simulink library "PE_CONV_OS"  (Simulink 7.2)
settings: Solver=ode45  SolverMode=SingleTasking  StartTime=0.0  StopTime=10.0  RelTol=1e-3
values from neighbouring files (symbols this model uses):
  C = 10e-3*1    (= 0.01)    [INIT_B6_2L_3Ph_IGBT_OS.m]    (also in INIT_B6_3L_3Ph_IGBT_OS.m; INIT_MMC_100L.m = 0.005; INIT_MMC_200L.m = 0.005; INIT_MMC_20L.m)
  FS = 900    [INIT_B6_2L_3Ph_IGBT_OS.m]    (also in INIT_B6_3L_3Ph_IGBT_OS.m; INIT_PWM_2L.m = 1000; INIT_PWM_3L.m = 1000; INIT_PWM_Con.m = 1000)
  LN = 2e-3    (= 0.002)    [INIT_PWM_2L.m]    (also in INIT_PWM_3L.m; INIT_PWM_Con.m; INIT_MMC_100L.m = 0.025; INIT_MMC_200L.m = 0.025)
  LS = 1e-3    (= 0.001)    [INIT_B6_2L_3Ph_IGBT_OS.m]    (also in INIT_B6_3L_3Ph_IGBT_OS.m; INIT_MMC_100L.m = 0.025; INIT_MMC_200L.m = 0.025; INIT_MMC_20L.m = 0.0025)
  LT = LN    (= 0.025)    [INIT_MMC_100L.m]    (also in INIT_MMC_200L.m; INIT_MMC_20L.m = 0.002; INIT_MMC_400L.m)
  Nc = 100    [INIT_MMC_100L.m]    (also in INIT_MMC_200L.m = 200; INIT_MMC_20L.m = 20; INIT_MMC_400L.m = 400)
  NT = sqrt(3)*340/400    [INIT_MMC_100L.m]    (also in INIT_MMC_200L.m; INIT_MMC_20L.m = sqrt(3); INIT_MMC_400L.m)
  Rg = 1e-3    (= 0.001)    [INIT_MMC_100L.m]    (also in INIT_MMC_200L.m; INIT_MMC_20L.m; INIT_MMC_400L.m)
  RN = 0.1    [INIT_PWM_2L.m]    (also in INIT_PWM_3L.m; INIT_PWM_Con.m; INIT_MMC_100L.m; INIT_MMC_200L.m)
  RT = RN    (= 0.1)    [INIT_MMC_100L.m]    (also in INIT_MMC_200L.m; INIT_MMC_20L.m; INIT_MMC_400L.m)
  UC0 = 600    [INIT_B6_2L_3Ph_IGBT_OS.m]    (also in INIT_B6_3L_3Ph_IGBT_OS.m = 500; INIT_MMC_100L.m = 6800; INIT_MMC_200L.m = 3400; INIT_MMC_20L.m = 5000)
undefined symbols (not defined in the file or in its folder): A, DT, FT, L, O1, O2, PHT, T, Td
libraries: simulink_extras x2
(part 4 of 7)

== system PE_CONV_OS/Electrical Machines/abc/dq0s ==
  a : Inport  OutDataType=sfix(16)  OutScaling=2^0
  b : Inport  Port=2  OutDataType=sfix(16)  OutScaling=2^0
  c : Inport  Port=3  OutDataType=sfix(16)  OutScaling=2^0
  Demux : Demux  Outputs=3
  K : Gain  Gain="2/3*[1   -.5   -.5;  0   sqrt(3)/2   -sqrt(3)/2;  .5    .5    .5]"  Multiplication=Matrix(K*u)  ParameterDataType=sfix(16)  ParameterScaling=2^0  OutDataType=sfix(16)  OutScaling=2^0
  Mux : Mux  Inputs=3
  d : Outport
  q : Outport  Port=2
  0 : Outport  Port=3
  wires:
  c/1 -> Mux/3
  b/1 -> Mux/2
  K/1 -> Demux/1
  Mux/1 -> K/1
  a/1 -> Mux/1
  Demux/1 -> d/1
  Demux/2 -> q/1
  Demux/3 -> 0/1

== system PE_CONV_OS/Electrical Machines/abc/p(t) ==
  Uabc : Inport
  Iabc : Inport  Port=2
  Fcn : Fcn  Expr=u(1)*u(4) + u(2)*u(5) + u(3)*u(6)
  Mux : Mux  Inputs=2
  Pt : Outport
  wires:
  Uabc/1 -> Mux/1
  Iabc/1 -> Mux/2
  Mux/1 -> Fcn/1
  Fcn/1 -> Pt/1

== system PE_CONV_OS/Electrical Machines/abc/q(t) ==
  Uabc : Inport
  Iabc : Inport  Port=2
  Fcn : Fcn  Expr="(  (u(2) - u(3))* u(4) + (u(3) - u(1))* u(5) + (u(1) - u(2))* u(6)  )/ sqrt(3)"
  Mux : Mux  Inputs=2
  qt : Outport
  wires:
  Uabc/1 -> Mux/1
  Iabc/1 -> Mux/2
  Mux/1 -> Fcn/1
  Fcn/1 -> qt/1

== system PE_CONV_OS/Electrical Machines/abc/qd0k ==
  a : Inport  OutDataType=sfix(16)  OutScaling=2^0
  b : Inport  Port=2  OutDataType=sfix(16)  OutScaling=2^0
  c : Inport  Port=3  OutDataType=sfix(16)  OutScaling=2^0
  th : Inport  Port=4  OutDataType=sfix(16)  OutScaling=2^0
  Demux : Demux  Outputs=3
  Fcn : Fcn  Expr=u(1)*cos(u(3)) - u(2)*sin(u(3))
  Fcn1 : Fcn  Expr=u(1)*sin(u(3)) + u(2)*cos(u(3))
  K : Gain  Gain="2/3*[1   -.5   -.5;  0   -sqrt(3)/2   sqrt(3)/2;  .5    .5    .5]"  Multiplication=Matrix(K*u)  ParameterDataType=sfix(16)  ParameterScaling=2^0  OutDataType=sfix(16)  OutScaling=2^0
  Mux : Mux  Inputs=3
  Mux1 : Mux  Inputs=3
  qk : Outport
  dk : Outport  Port=2
  0k : Outport  Port=3
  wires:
  Demux/2 -> Mux1/2
  Demux/1 -> Mux1/1
  Demux/3 -> 0k/1
  th/1 -> Mux1/3
  Fcn1/1 -> dk/1
  Fcn/1 -> qk/1
  Mux1/1 -> Fcn/1, Fcn1/1
  a/1 -> Mux/1
  Mux/1 -> K/1
  K/1 -> Demux/1
  b/1 -> Mux/2
  c/1 -> Mux/3

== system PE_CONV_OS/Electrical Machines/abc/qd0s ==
  a : Inport  OutDataType=sfix(16)  OutScaling=2^0
  b : Inport  Port=2  OutDataType=sfix(16)  OutScaling=2^0
  c : Inport  Port=3  OutDataType=sfix(16)  OutScaling=2^0
  Demux : Demux  Outputs=3
  K : Gain  Gain="2/3*[1   -.5   -.5;  0   -sqrt(3)/2   sqrt(3)/2;  .5    .5    .5]"  Multiplication=Matrix(K*u)  ParameterDataType=sfix(16)  ParameterScaling=2^0  OutDataType=sfix(16)  OutScaling=2^0
  Mux : Mux  Inputs=3
  q : Outport
  d : Outport  Port=2
  0 : Outport  Port=3
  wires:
  Demux/3 -> 0/1
  Demux/2 -> d/1
  Demux/1 -> q/1
  a/1 -> Mux/1
  Mux/1 -> K/1
  K/1 -> Demux/1
  b/1 -> Mux/2
  c/1 -> Mux/3

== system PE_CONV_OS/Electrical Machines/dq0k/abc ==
  dk : Inport  OutDataType=sfix(16)  OutScaling=2^0
  qk : Inport  Port=2  OutDataType=sfix(16)  OutScaling=2^0
  0k : Inport  Port=3  OutDataType=sfix(16)  OutScaling=2^0
  th : Inport  Port=4  OutDataType=sfix(16)  OutScaling=2^0
  Demux : Demux  Outputs=3
  Fcn : Fcn  Expr=u(1)*cos(u(3)) - u(2)*sin(u(3))
  Fcn1 : Fcn  Expr=u(1)*sin(u(3)) + u(2)*cos(u(3))
  K : Gain  Gain="[1   0  1 ;  -.5   sqrt(3)/2    1 ;  -.5    -sqrt(3)/2    1]"  Multiplication=Matrix(K*u)  ParameterDataType=sfix(16)  ParameterScaling=2^0  OutDataType=sfix(16)  OutScaling=2^0
  Mux : Mux  Inputs=3
  Mux1 : Mux  Inputs=3
  a : Outport
  b : Outport  Port=2
  c : Outport  Port=3
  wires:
  0k/1 -> Mux1/3
  th/1 -> Mux/3
  Demux/3 -> c/1
  Demux/2 -> b/1
  Demux/1 -> a/1
  Fcn1/1 -> Mux1/2
  Fcn/1 -> Mux1/1
  Mux1/1 -> K/1
  K/1 -> Demux/1
  Mux/1 -> Fcn1/1, Fcn/1
  qk/1 -> Mux/2
  dk/1 -> Mux/1

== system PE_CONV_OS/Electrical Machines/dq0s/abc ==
  d : Inport  OutDataType=sfix(16)  OutScaling=2^0
  q : Inport  Port=2  OutDataType=sfix(16)  OutScaling=2^0
  0 : Inport  Port=3  OutDataType=sfix(16)  OutScaling=2^0
  Demux : Demux  Outputs=3
  K : Gain  Gain="[1   0  1;  -.5   sqrt(3)/2   1;  -.5    -sqrt(3)/2  1]"  Multiplication=Matrix(K*u)  ParameterDataType=sfix(16)  ParameterScaling=2^0  OutDataType=sfix(16)  OutScaling=2^0
  Mux : Mux  Inputs=3
  a : Outport
  b : Outport  Port=2
  c : Outport  Port=3
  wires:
  q/1 -> Mux/2
  K/1 -> Demux/1
  Mux/1 -> K/1
  Demux/2 -> b/1
  Demux/3 -> c/1
  0/1 -> Mux/3
  d/1 -> Mux/1
  Demux/1 -> a/1

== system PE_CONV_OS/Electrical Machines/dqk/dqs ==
  dk : Inport  OutDataType=sfix(16)  OutScaling=2^0
  qk : Inport  Port=2  OutDataType=sfix(16)  OutScaling=2^0
  0k : Inport  Port=3  OutDataType=sfix(16)  OutScaling=2^0
  th : Inport  Port=4  OutDataType=sfix(16)  OutScaling=2^0
  Fcn : Fcn  Expr=u(1)*cos(u(3)) - u(2)*sin(u(3))
  Fcn1 : Fcn  Expr=u(1)*sin(u(3)) + u(2)*cos(u(3))
  Mux : Mux  Inputs=3
  ds : Outport
  qs : Outport  Port=2
  0s : Outport  Port=3
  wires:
  Fcn1/1 -> qs/1
  Fcn/1 -> ds/1
  Mux/1 -> Fcn1/1, Fcn/1
  qk/1 -> Mux/2
  dk/1 -> Mux/1
  th/1 -> Mux/3
  0k/1 -> 0s/1

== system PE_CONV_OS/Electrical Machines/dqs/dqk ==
  ds : Inport  OutDataType=sfix(16)  OutScaling=2^0
  qs : Inport  Port=2  OutDataType=sfix(16)  OutScaling=2^0
  0s : Inport  Port=3  OutDataType=sfix(16)  OutScaling=2^0
  th : Inport  Port=4  OutDataType=sfix(16)  OutScaling=2^0
  Fcn : Fcn  Expr=u(1)*cos(u(3)) + u(2)*sin(u(3))
  Fcn1 : Fcn  Expr=-u(1)*sin(u(3)) + u(2)*cos(u(3))
  Mux : Mux  Inputs=3
  dk : Outport
  qk : Outport  Port=2
  0k : Outport  Port=3
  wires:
  Fcn1/1 -> qk/1
  Fcn/1 -> dk/1
  Mux/1 -> Fcn1/1, Fcn/1
  qs/1 -> Mux/2
  ds/1 -> Mux/1
  th/1 -> Mux/3
  0s/1 -> 0k/1

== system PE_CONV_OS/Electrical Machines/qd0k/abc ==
  qk : Inport  OutDataType=sfix(16)  OutScaling=2^0
  dk : Inport  Port=2  OutDataType=sfix(16)  OutScaling=2^0
  0k : Inport  Port=3  OutDataType=sfix(16)  OutScaling=2^0
  th : Inport  Port=4  OutDataType=sfix(16)  OutScaling=2^0
  Demux : Demux  Outputs=3
  Fcn : Fcn  Expr=u(1)*cos(u(3)) + u(2)*sin(u(3))
  Fcn1 : Fcn  Expr=-u(1)*sin(u(3)) + u(2)*cos(u(3))
  K : Gain  Gain="[1   0  1 ;  -.5   -sqrt(3)/2    1 ;  -.5    sqrt(3)/2    1]"  Multiplication=Matrix(K*u)  ParameterDataType=sfix(16)  ParameterScaling=2^0  OutDataType=sfix(16)  OutScaling=2^0
  Mux : Mux  Inputs=3
  Mux1 : Mux  Inputs=3
  a : Outport
  b : Outport  Port=2
  c : Outport  Port=3
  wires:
  0k/1 -> Mux1/3
  th/1 -> Mux/3
  Demux/3 -> c/1
  Demux/2 -> b/1
  Demux/1 -> a/1
  Fcn1/1 -> Mux1/2
  Fcn/1 -> Mux1/1
  Mux1/1 -> K/1
  K/1 -> Demux/1
  Mux/1 -> Fcn1/1, Fcn/1
  dk/1 -> Mux/2
  qk/1 -> Mux/1

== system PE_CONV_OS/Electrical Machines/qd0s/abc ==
  q : Inport  OutDataType=sfix(16)  OutScaling=2^0
  d : Inport  Port=2  OutDataType=sfix(16)  OutScaling=2^0
  0 : Inport  Port=3  OutDataType=sfix(16)  OutScaling=2^0
  Demux : Demux  Outputs=3
  K : Gain  Gain="[1   0  1;  -.5   -sqrt(3)/2   1;  -.5    sqrt(3)/2  1]"  Multiplication=Matrix(K*u)  ParameterDataType=sfix(16)  ParameterScaling=2^0  OutDataType=sfix(16)  OutScaling=2^0
  Mux : Mux  Inputs=3
  a : Outport
  b : Outport  Port=2
  c : Outport  Port=3
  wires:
  d/1 -> Mux/2
  K/1 -> Demux/1
  Mux/1 -> K/1
  Demux/2 -> b/1
  Demux/3 -> c/1
  0/1 -> Mux/3
  q/1 -> Mux/1
  Demux/1 -> a/1

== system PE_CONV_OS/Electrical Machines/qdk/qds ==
  qk : Inport  OutDataType=sfix(16)  OutScaling=2^0
  dk : Inport  Port=2  OutDataType=sfix(16)  OutScaling=2^0
  0k : Inport  Port=3  OutDataType=sfix(16)  OutScaling=2^0
  th : Inport  Port=4  OutDataType=sfix(16)  OutScaling=2^0
  Fcn : Fcn  Expr=u(1)*cos(u(3)) + u(2)*sin(u(3))
  Fcn1 : Fcn  Expr=-u(1)*sin(u(3)) + u(2)*cos(u(3))
  Mux : Mux  Inputs=3
  qs : Outport
  ds : Outport  Port=2
  0s : Outport  Port=3
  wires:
  Fcn1/1 -> ds/1
  Fcn/1 -> qs/1
  Mux/1 -> Fcn1/1, Fcn/1
  dk/1 -> Mux/2
  qk/1 -> Mux/1
  th/1 -> Mux/3
  0k/1 -> 0s/1

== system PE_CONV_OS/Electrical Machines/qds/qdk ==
  qs : Inport  OutDataType=sfix(16)  OutScaling=2^0
  ds : Inport  Port=2  OutDataType=sfix(16)  OutScaling=2^0
  0s : Inport  Port=3  OutDataType=sfix(16)  OutScaling=2^0
  th : Inport  Port=4  OutDataType=sfix(16)  OutScaling=2^0
  Fcn : Fcn  Expr=u(1)*cos(u(3)) - u(2)*sin(u(3))
  Fcn1 : Fcn  Expr=u(1)*sin(u(3)) + u(2)*cos(u(3))
  Mux : Mux  Inputs=3
  qk : Outport
  dk : Outport  Port=2
  0k : Outport  Port=3
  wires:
  Fcn1/1 -> dk/1
  Fcn/1 -> qk/1
  Mux/1 -> Fcn1/1, Fcn/1
  ds/1 -> Mux/2
  qs/1 -> Mux/1
  0s/1 -> 0k/1
  th/1 -> Mux/3

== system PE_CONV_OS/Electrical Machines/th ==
  abc : Inport
  C : ComplexToMagnitudeAngle
  Demux : Demux  Outputs=3
  K : Gain  Gain="2/3*[1   -.5   -.5;  0   sqrt(3)/2   -sqrt(3)/2;  .5    .5    .5]"  Multiplication=Matrix(K*u)
  R : RealImagToComplex
  |u| : Outport
  th : Outport  Port=2
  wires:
  C/2 -> th/1
  R/1 -> C/1
  Demux/2 -> R/2
  Demux/1 -> R/1
  abc/1 -> K/1
  K/1 -> Demux/1
  C/1 -> |u|/1

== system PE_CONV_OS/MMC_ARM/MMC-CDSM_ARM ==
  In : Inport  OutDataType=sfix(16)  OutScaling=2^0
  MMC_CDSM_ARM : S-Function  FunctionName=s_MMC_CDSM_ARM  Parameters="[C   UC0   Nc]"  EnableBusSupport=off
  VCs : Outport  OutDataType=sfix(16)  OutScaling=2^0
  IC1 : Outport  Port=2  OutDataType=sfix(16)  OutScaling=2^0
  IT1,ID1,VT1 : Outport  Port=3  OutDataType=sfix(16)  OutScaling=2^0
  IT2,ID2,VT2 : Outport  Port=4  OutDataType=sfix(16)  OutScaling=2^0
  V_arm : Outport  Port=5  OutDataType=sfix(16)  OutScaling=2^0
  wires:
  MMC_CDSM_ARM/5 -> V_arm/1
  MMC_CDSM_ARM/4 -> IT2,ID2,VT2/1
  MMC_CDSM_ARM/3 -> IT1,ID1,VT1/1
  MMC_CDSM_ARM/2 -> IC1/1
  MMC_CDSM_ARM/1 -> VCs/1
  In/1 -> MMC_CDSM_ARM/1

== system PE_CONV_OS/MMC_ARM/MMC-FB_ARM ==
  In : Inport  OutDataType=sfix(16)  OutScaling=2^0
  MMC_FB_ARM : S-Function  FunctionName=s_MMC_FB_ARM  Parameters="[C   UC0   Nc]"  EnableBusSupport=off
  VCs : Outport  OutDataType=sfix(16)  OutScaling=2^0
  IC1 : Outport  Port=2  OutDataType=sfix(16)  OutScaling=2^0
  IT1,ID1,VT1 : Outport  Port=3  OutDataType=sfix(16)  OutScaling=2^0
  IT2,ID2,VT2 : Outport  Port=4  OutDataType=sfix(16)  OutScaling=2^0
  V_arm : Outport  Port=5  OutDataType=sfix(16)  OutScaling=2^0
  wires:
  In/1 -> MMC_FB_ARM/1
  MMC_FB_ARM/1 -> VCs/1
  MMC_FB_ARM/2 -> IC1/1
  MMC_FB_ARM/3 -> IT1,ID1,VT1/1
  MMC_FB_ARM/4 -> IT2,ID2,VT2/1
  MMC_FB_ARM/5 -> V_arm/1

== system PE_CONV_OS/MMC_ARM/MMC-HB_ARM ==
  In : Inport  OutDataType=sfix(16)  OutScaling=2^0
  MMC_HB_ARM : S-Function  FunctionName=s_MMC_HB_ARM  Parameters="[C   UC0   Nc]"  EnableBusSupport=off
  VCs : Outport  OutDataType=sfix(16)  OutScaling=2^0
  IC1 : Outport  Port=2  OutDataType=sfix(16)  OutScaling=2^0
  IT1,ID1,VT1 : Outport  Port=3  OutDataType=sfix(16)  OutScaling=2^0
  IT2,ID2,VT2 : Outport  Port=4  OutDataType=sfix(16)  OutScaling=2^0
  V_arm : Outport  Port=5  OutDataType=sfix(16)  OutScaling=2^0
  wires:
  MMC_HB_ARM/5 -> V_arm/1
  MMC_HB_ARM/4 -> IT2,ID2,VT2/1
  MMC_HB_ARM/3 -> IT1,ID1,VT1/1
  MMC_HB_ARM/2 -> IC1/1
  MMC_HB_ARM/1 -> VCs/1
  In/1 -> MMC_HB_ARM/1

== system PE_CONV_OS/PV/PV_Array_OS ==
  G : Inport
  Temp : Inport  Port=2
  ILd : Inport  Port=3
  Mux : Mux  Inputs=3
  t_PV_Array_OS : S-Function  FunctionName=s_PV_Array_OS  Parameters="[Isc0  Ud0  Ki  Kv  n    RS  RP NC  NMs NMp C  vC0  RL]"  EnableBusSupport=off
  PV_I : Outport
  PV_V : Outport  Port=2
  C_I : Outport  Port=3
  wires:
  Mux/1 -> t_PV_Array_OS/1
  G/1 -> Mux/1
  Temp/1 -> Mux/2
  ILd/1 -> Mux/3
  t_PV_Array_OS/1 -> PV_I/1
  t_PV_Array_OS/2 -> PV_V/1
  t_PV_Array_OS/3 -> C_I/1

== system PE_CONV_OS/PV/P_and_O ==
  V : Inport  OutDataType=sfix(16)  OutScaling=2^0
  I : Inport  Port=2  OutDataType=sfix(16)  OutScaling=2^0
  Add : Sum  Inputs=+-  OutDataType=sfix(16)  OutScaling=2^-10
  Add1 : Sum  Inputs=+-  OutDataType=sfix(16)  OutScaling=2^-10
  Add2 : Sum  OutDataType=sfix(16)  OutScaling=2^-10
  Constant : Constant  Value=-1  OutDataType=sfix(16)  OutScaling=2^0
  Constant1 : Constant  OutDataType=sfix(16)  OutScaling=2^0
  DeltaD : Constant  Value=DeltaD  OutDataType=sfix(16)  OutScaling=2^0
  M : Memory
  M1 : Memory
  M2 : Memory  Orientation=left
  Mul{,1..3} (4 alike) : Product  Inputs=**  OutDataType=sfix(16)  OutScaling=2^-10
  Sat : Saturate  UpperLimit=1  LowerLimit=0  OutDataType=sfix(16)  OutScaling=2^0
  Switch : Switch  OutDataType=sfix(16)  OutScaling=2^0
  TF : TransferFcn  Denominator=[1e-4 1]
  D : Outport  OutDataType=sfix(16)  OutScaling=2^0
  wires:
  I/1 -> Mul/2, M1/1
  V/1 -> Mul/1, M/1, Add1/1
  M/1 -> Mul1/1, Add1/2
  M1/1 -> Mul1/2
  Mul/1 -> Add/1
  Mul1/1 -> Add/2
  Add/1 -> Mul2/1
  Add1/1 -> Mul2/2
  Mul2/1 -> Switch/2
  Constant/1 -> Switch/1
  Constant1/1 -> Switch/3
  Switch/1 -> Mul3/2
  DeltaD/1 -> Mul3/1
  Mul3/1 -> Add2/1
  Add2/1 -> M2/1, TF/1
  M2/1 -> Add2/2
  TF/1 -> Sat/1
  Sat/1 -> D/1

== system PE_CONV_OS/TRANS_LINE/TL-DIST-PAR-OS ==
  V_In : Inport  OutDataType=sfix(16)  OutScaling=2^0
  I_Load : Inport  Port=2  OutDataType=sfix(16)  OutScaling=2^0
  Mux : Mux  Inputs=2
  TL-DIST-PAR-OS : S-Function  FunctionName=s_TL_DIST_PAR_OS  Parameters=[L C R TL RS ]  EnableBusSupport=off
  TL_V_IN : Outport  OutDataType=sfix(16)  OutScaling=2^0
  TL_V_OUT : Outport  Port=2  OutDataType=sfix(16)  OutScaling=2^0
  TL_I_IN : Outport  Port=3  OutDataType=sfix(16)  OutScaling=2^0
  TL_I_OUT : Outport  Port=4  OutDataType=sfix(16)  OutScaling=2^0
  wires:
  TL-DIST-PAR-OS/4 -> TL_I_OUT/1
  Mux/1 -> TL-DIST-PAR-OS/1
  V_In/1 -> Mux/1
  I_Load/1 -> Mux/2
  TL-DIST-PAR-OS/1 -> TL_V_IN/1
  TL-DIST-PAR-OS/2 -> TL_V_OUT/1
  TL-DIST-PAR-OS/3 -> TL_I_IN/1

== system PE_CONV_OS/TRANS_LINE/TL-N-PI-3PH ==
  VS_ABC : Inport  OutDataType=sfix(16)  OutScaling=2^0
  IL12 : Inport  Port=2  OutDataType=sfix(16)  OutScaling=2^0
  Mux : Mux  Inputs="[3  3]"
  TL3PH_OS : S-Function  FunctionName=s_TL_N_PI_3PH_OS  Parameters=[R L C TL N RS LS ]  EnableBusSupport=off
  IABC : Outport  OutDataType=sfix(16)  OutScaling=2^0
  Iabc : Outport  Port=2  OutDataType=sfix(16)  OutScaling=2^0
  VABC : Outport  Port=3  OutDataType=sfix(16)  OutScaling=2^0
  Vabc : Outport  Port=4  OutDataType=sfix(16)  OutScaling=2^0
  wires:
  TL3PH_OS/3 -> VABC/1
  TL3PH_OS/2 -> Iabc/1
  TL3PH_OS/1 -> IABC/1
  IL12/1 -> Mux/2
  VS_ABC/1 -> Mux/1
  Mux/1 -> TL3PH_OS/1
  TL3PH_OS/4 -> Vabc/1

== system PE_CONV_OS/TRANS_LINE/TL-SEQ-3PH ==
  VS_ABC : Inport  OutDataType=sfix(16)  OutScaling=2^0
  IL12 : Inport  Port=2  OutDataType=sfix(16)  OutScaling=2^0
  Mux : Mux  Inputs="[3  3]"
  TL3PH_DP_OS : S-Function  FunctionName=s_TL_N_PI_3PH_SEQ_OS  Parameters="[R1 R0  L1  L0 C1 C0  TL NS  RS LS ]"  EnableBusSupport=off
  IABC : Outport  OutDataType=sfix(16)  OutScaling=2^0
  Iabc : Outport  Port=2  OutDataType=sfix(16)  OutScaling=2^0
  VABC : Outport  Port=3  OutDataType=sfix(16)  OutScaling=2^0
  Vabc : Outport  Port=4  OutDataType=sfix(16)  OutScaling=2^0
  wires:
  TL3PH_DP_OS/3 -> VABC/1
  TL3PH_DP_OS/2 -> Iabc/1
  TL3PH_DP_OS/1 -> IABC/1
  IL12/1 -> Mux/2
  VS_ABC/1 -> Mux/1
  Mux/1 -> TL3PH_DP_OS/1
  TL3PH_DP_OS/4 -> Vabc/1

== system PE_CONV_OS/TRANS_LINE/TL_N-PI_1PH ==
  V_In : Inport  OutDataType=sfix(16)  OutScaling=2^0
  I_Load : Inport  Port=2  OutDataType=sfix(16)  OutScaling=2^0
  Mux : Mux  Inputs=2
  TL-N-PI-SECTIONS : S-Function  FunctionName=s_TL_N_PI_OS  Parameters=[L C R TL N R1 ]  EnableBusSupport=off
  TL_V_IN : Outport  OutDataType=sfix(16)  OutScaling=2^0
  TL_V_OUT : Outport  Port=2  OutDataType=sfix(16)  OutScaling=2^0
  TL_I_IN : Outport  Port=3  OutDataType=sfix(16)  OutScaling=2^0
  TL_I_OUT : Outport  Port=4  OutDataType=sfix(16)  OutScaling=2^0
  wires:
  TL-N-PI-SECTIONS/3 -> TL_I_IN/1
  TL-N-PI-SECTIONS/2 -> TL_V_OUT/1
  TL-N-PI-SECTIONS/1 -> TL_V_IN/1
  I_Load/1 -> Mux/2
  V_In/1 -> Mux/1
  Mux/1 -> TL-N-PI-SECTIONS/1
  TL-N-PI-SECTIONS/4 -> TL_I_OUT/1

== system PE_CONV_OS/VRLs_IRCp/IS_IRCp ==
  IS : Inport
  IL : Inport  Port=2
  IRCp : S-Function  FunctionName=s_IS_IRCp_OS  Parameters=[R, C, VC0, RCs]  EnableBusSupport=off
  Mux : Mux  Inputs=2
  iC : Outport
  vC : Outport  Port=2
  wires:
  IL/1 -> Mux/2
  IS/1 -> Mux/1
  Mux/1 -> IRCp/1
  IRCp/2 -> vC/1
  IRCp/1 -> iC/1

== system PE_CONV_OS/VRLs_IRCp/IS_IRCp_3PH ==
  IS123 : Inport
  IL123 : Inport  Port=2
  IRCp_3PH : S-Function  FunctionName=s_IS_IRCp_3PH_OS  Parameters=[R,C,RCs]  EnableBusSupport=off
  Mux : Mux  Inputs="[3  3]"
  iC123 : Outport
  VC123 : Outport  Port=2
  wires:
  IRCp_3PH/2 -> VC123/1
  IL123/1 -> Mux/2
  IS123/1 -> Mux/1
  Mux/1 -> IRCp_3PH/1
  IRCp_3PH/1 -> iC123/1

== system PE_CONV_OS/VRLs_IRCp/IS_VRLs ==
  VS : Inport
  E : Inport  Port=2
  Mux : Mux  Inputs=2
  RL : S-Function  FunctionName=s_IS_VRLs_OS  Parameters=[R, L, IL0, RLp]  EnableBusSupport=off
  iL : Outport
  vL : Outport  Port=2
  vR : Outport  Port=3
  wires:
  Mux/1 -> RL/1
  E/1 -> Mux/2
  VS/1 -> Mux/1
  RL/1 -> iL/1
  RL/2 -> vL/1
  RL/3 -> vR/1

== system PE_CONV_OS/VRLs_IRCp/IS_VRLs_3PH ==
  VS123 : Inport
  E123 : Inport  Port=2
  Mux : Mux  Inputs="[3  3]"
  RL : S-Function  FunctionName=s_IS_VRLs_3PH_OS  Parameters=[R, L, RLp]  EnableBusSupport=off
  iL123 : Outport
  VL123 : Outport  Port=2
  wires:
  RL/2 -> VL123/1
  RL/1 -> iL123/1
  Mux/1 -> RL/1
  VS123/1 -> Mux/1
  E123/1 -> Mux/2

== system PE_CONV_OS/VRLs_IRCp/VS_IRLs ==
  VS : Inport
  IL : Inport  Port=2
  IRp : S-Function  FunctionName=s_VS_IRp_OS  Parameters=[R]  EnableBusSupport=off
  Mux : Mux  Inputs=2
  iR : Outport
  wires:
  IRp/1 -> iR/1
  Mux/1 -> IRp/1
  VS/1 -> Mux/1
  IL/1 -> Mux/2

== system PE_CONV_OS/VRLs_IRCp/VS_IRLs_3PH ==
  VS123 : Inport
  IL123 : Inport  Port=2
  IRLs_3PH : S-Function  FunctionName=s_VS_IRLs_3PH_OS  Parameters=[R L]  EnableBusSupport=off
  Mux : Mux  Inputs="[3  3]"
  iR123 : Outport
  VO123 : Outport  Port=2
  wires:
  IRLs_3PH/1 -> iR123/1
  Mux/1 -> IRLs_3PH/1
  VS123/1 -> Mux/1
  IL123/1 -> Mux/2
  IRLs_3PH/2 -> VO123/1

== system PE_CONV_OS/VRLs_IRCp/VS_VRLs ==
  VS : Inport
  E : Inport  Port=2
  Mux : Mux  Inputs=2
  RL : S-Function  FunctionName=s_VS_VRLs_OS  Parameters=[R, L, IL0, RLp]  EnableBusSupport=off
  iL : Outport
  vL : Outport  Port=2
  vR : Outport  Port=3
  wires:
  RL/3 -> vR/1
  RL/2 -> vL/1
  RL/1 -> iL/1
  VS/1 -> Mux/1
  E/1 -> Mux/2
  Mux/1 -> RL/1

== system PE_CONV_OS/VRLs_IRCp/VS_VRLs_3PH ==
  VS123 : Inport
  E123 : Inport  Port=2
  Mux : Mux  Inputs="[3  3]"
  RL : S-Function  FunctionName=s_VS_VRLs_3PH_OS  Parameters=[R, L, RLp]  EnableBusSupport=off
  iL123 : Outport
  VL123 : Outport  Port=2
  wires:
  E123/1 -> Mux/2
  VS123/1 -> Mux/1
  Mux/1 -> RL/1
  RL/1 -> iL123/1
  RL/2 -> VL123/1

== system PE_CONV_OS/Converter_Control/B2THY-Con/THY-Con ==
  In1 : Inport  OutDataType=sfix(16)  OutScaling=2^0
  DT : DataTypeConversion
  DT1 : DataTypeConversion
  DT2 : DataTypeConversion
  Fcn : Fcn  Expr="(u  > 0.9999)*2 + (u<=0.9999)*u"
  Relay : Relay  OutDataType=sfix(16)  OutScaling=2^0
  Sine Wave1 : Sin  Frequency=F*2*pi  Phase=PH*pi/180  SampleTime=0
  Sum1 : Sum  Inputs=-+  OutDataType=sfix(16)  OutScaling=2^0
  TonDelay : Subsystem  mask(TonDelay){DT=TD}
      mask prompts: DT "Dead Time"
      mask help: Turn on dead time to protect against short circuit of the converter leg
  XOR : Logic  Operator=XOR
  Out1 : Outport
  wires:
  In1/1 -> Sum1/2
  Sum1/1 -> Relay/1
  TonDelay/1(s1d) -> DT1/1
  Relay/1 -> TonDelay/1(s1), DT2/1
  XOR/1 -> DT/1
  Sine Wave1/1 -> Fcn/1
  Fcn/1 -> Sum1/1
  DT/1 -> Out1/1
  DT1/1 -> XOR/1
  DT2/1 -> XOR/2

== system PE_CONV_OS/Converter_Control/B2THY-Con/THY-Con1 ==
  In1 : Inport  OutDataType=sfix(16)  OutScaling=2^0
  DT : DataTypeConversion
  DT1 : DataTypeConversion
  DT2 : DataTypeConversion
  Fcn : Fcn  Expr="(u  > 0.9999)*2 + (u<=0.9999)*u"
  Relay : Relay  OutDataType=sfix(16)  OutScaling=2^0
  Sine Wave1 : Sin  Frequency=F*2*pi  Phase=PH*pi/180  SampleTime=0
  Sum1 : Sum  Inputs=-+  OutDataType=sfix(16)  OutScaling=2^0
  TonDelay : Subsystem  mask(TonDelay){DT=TD}
      mask prompts: DT "Dead Time"
      mask help: Turn on dead time to protect against short circuit of the converter leg
  XOR : Logic  Operator=XOR
  Out1 : Outport
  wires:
  Fcn/1 -> Sum1/1
  Sine Wave1/1 -> Fcn/1
  XOR/1 -> DT/1
  Relay/1 -> TonDelay/1(s1), DT2/1
  TonDelay/1(s1d) -> DT1/1
  Sum1/1 -> Relay/1
  In1/1 -> Sum1/2
  DT/1 -> Out1/1
  DT1/1 -> XOR/1
  DT2/1 -> XOR/2

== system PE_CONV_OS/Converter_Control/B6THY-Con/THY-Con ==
  In1 : Inport  OutDataType=sfix(16)  OutScaling=2^0
  DT1 : DataTypeConversion
  DT2 : DataTypeConversion
  Fcn : Fcn  Expr="(u  > 0.9999)*2 + (u<=0.9999)*u"
  Relay : Relay  OutDataType=sfix(16)  OutScaling=2^0
  Sine Wave1 : Sin  Frequency=F*2*pi  Phase=PH*pi/180  SampleTime=0
  Sum1 : Sum  Inputs=-+  OutDataType=sfix(16)  OutScaling=2^0
  TonDelay : Subsystem  mask(TonDelay){DT=TD}
      mask prompts: DT "Dead Time"
      mask help: Turn on dead time to protect against short circuit of the converter leg
  XOR : Logic  Operator=XOR
  Out1 : Outport
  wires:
  In1/1 -> Sum1/2
  Sum1/1 -> Relay/1
  TonDelay/1(s1d) -> DT1/1
  Relay/1 -> TonDelay/1(s1), DT2/1
  XOR/1 -> Out1/1
  Sine Wave1/1 -> Fcn/1
  Fcn/1 -> Sum1/1
  DT1/1 -> XOR/1
  DT2/1 -> XOR/2

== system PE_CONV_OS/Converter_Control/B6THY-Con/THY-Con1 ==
  In1 : Inport  OutDataType=sfix(16)  OutScaling=2^0
  DT : DataTypeConversion
  DT1 : DataTypeConversion
  Fcn : Fcn  Expr="(u  > 0.9999)*2 + (u<=0.9999)*u"
  Relay : Relay  OutDataType=sfix(16)  OutScaling=2^0
  Sine Wave1 : Sin  Frequency=F*2*pi  Phase=PH*pi/180  SampleTime=0
  Sum1 : Sum  Inputs=-+  OutDataType=sfix(16)  OutScaling=2^0
  TonDelay : Subsystem  mask(TonDelay){DT=TD}
      mask prompts: DT "Dead Time"
      mask help: Turn on dead time to protect against short circuit of the converter leg
  XOR : Logic  Operator=XOR
  Out1 : Outport
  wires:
  Fcn/1 -> Sum1/1
  Sine Wave1/1 -> Fcn/1
  XOR/1 -> Out1/1
  Relay/1 -> TonDelay/1(s1), DT1/1
  TonDelay/1(s1d) -> DT/1
  Sum1/1 -> Relay/1
  In1/1 -> Sum1/2
  DT/1 -> XOR/1
  DT1/1 -> XOR/2

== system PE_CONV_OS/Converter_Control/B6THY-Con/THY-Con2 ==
  In1 : Inport  OutDataType=sfix(16)  OutScaling=2^0
  DT : DataTypeConversion
  DT1 : DataTypeConversion
  Fcn : Fcn  Expr="(u  > 0.9999)*2 + (u<=0.9999)*u"
  Relay : Relay  OutDataType=sfix(16)  OutScaling=2^0
  Sine Wave1 : Sin  Frequency=F*2*pi  Phase=PH*pi/180  SampleTime=0
  Sum1 : Sum  Inputs=-+  OutDataType=sfix(16)  OutScaling=2^0
  TonDelay : Subsystem  mask(TonDelay){DT=TD}
      mask prompts: DT "Dead Time"
      mask help: Turn on dead time to protect against short circuit of the converter leg
  XOR : Logic  Operator=XOR
  Out1 : Outport
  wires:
  In1/1 -> Sum1/2
  Sum1/1 -> Relay/1
  TonDelay/1(s1d) -> DT/1
  Relay/1 -> TonDelay/1(s1), DT1/1
  XOR/1 -> Out1/1
  Sine Wave1/1 -> Fcn/1
  Fcn/1 -> Sum1/1
  DT/1 -> XOR/1
  DT1/1 -> XOR/2

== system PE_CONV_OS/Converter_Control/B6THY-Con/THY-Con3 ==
  In1 : Inport  OutDataType=sfix(16)  OutScaling=2^0
  DT : DataTypeConversion
  DT1 : DataTypeConversion
  Fcn : Fcn  Expr="(u  > 0.9999)*2 + (u<=0.9999)*u"
  Relay : Relay  OutDataType=sfix(16)  OutScaling=2^0
  Sine Wave1 : Sin  Frequency=F*2*pi  Phase=PH*pi/180  SampleTime=0
  Sum1 : Sum  Inputs=-+  OutDataType=sfix(16)  OutScaling=2^0
  TonDelay : Subsystem  mask(TonDelay){DT=TD}
      mask prompts: DT "Dead Time"
      mask help: Turn on dead time to protect against short circuit of the converter leg
  XOR : Logic  Operator=XOR
  Out1 : Outport
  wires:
  Fcn/1 -> Sum1/1
  Sine Wave1/1 -> Fcn/1
  XOR/1 -> Out1/1
  Relay/1 -> TonDelay/1(s1), DT1/1
  TonDelay/1(s1d) -> DT/1
  Sum1/1 -> Relay/1
  In1/1 -> Sum1/2
  DT/1 -> XOR/1
  DT1/1 -> XOR/2

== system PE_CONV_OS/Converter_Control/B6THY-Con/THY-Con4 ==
  In1 : Inport  OutDataType=sfix(16)  OutScaling=2^0
  DT : DataTypeConversion
  DT1 : DataTypeConversion
  Fcn : Fcn  Expr="(u  > 0.9999)*2 + (u<=0.9999)*u"
  Relay : Relay  OutDataType=sfix(16)  OutScaling=2^0
  Sine Wave1 : Sin  Frequency=F*2*pi  Phase=PH*pi/180  SampleTime=0
  Sum1 : Sum  Inputs=-+  OutDataType=sfix(16)  OutScaling=2^0
  TonDelay : Subsystem  mask(TonDelay){DT=TD}
      mask prompts: DT "Dead Time"
      mask help: Turn on dead time to protect against short circuit of the converter leg
  XOR : Logic  Operator=XOR
  Out1 : Outport
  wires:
  In1/1 -> Sum1/2
  Sum1/1 -> Relay/1
  TonDelay/1(s1d) -> DT/1
  Relay/1 -> TonDelay/1(s1), DT1/1
  XOR/1 -> Out1/1
  Sine Wave1/1 -> Fcn/1
  Fcn/1 -> Sum1/1
  DT/1 -> XOR/1
  DT1/1 -> XOR/2

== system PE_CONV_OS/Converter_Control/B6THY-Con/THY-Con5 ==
  In1 : Inport  OutDataType=sfix(16)  OutScaling=2^0
  DT : DataTypeConversion
  DT1 : DataTypeConversion
  Fcn : Fcn  Expr="(u  > 0.9999)*2 + (u<=0.9999)*u"
  Relay : Relay  OutDataType=sfix(16)  OutScaling=2^0
  Sine Wave1 : Sin  Frequency=F*2*pi  Phase=PH*pi/180  SampleTime=0
  Sum1 : Sum  Inputs=-+  OutDataType=sfix(16)  OutScaling=2^0
  TonDelay : Subsystem  mask(TonDelay){DT=TD}
      mask prompts: DT "Dead Time"
      mask help: Turn on dead time to protect against short circuit of the converter leg
  XOR : Logic  Operator=XOR
  Out1 : Outport
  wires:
  Fcn/1 -> Sum1/1
  Sine Wave1/1 -> Fcn/1
  XOR/1 -> Out1/1
  Relay/1 -> TonDelay/1(s1), DT1/1
  TonDelay/1(s1d) -> DT/1
  Sum1/1 -> Relay/1
  In1/1 -> Sum1/2
  DT/1 -> XOR/1
  DT1/1 -> XOR/2

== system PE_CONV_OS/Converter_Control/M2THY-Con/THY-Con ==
  In1 : Inport  OutDataType=sfix(16)  OutScaling=2^0
  DT : DataTypeConversion
  DT1 : DataTypeConversion
  DT2 : DataTypeConversion
  Fcn : Fcn  Expr="(u  > 0.9999)*2 + (u<=0.9999)*u"
  Relay : Relay  OutDataType=sfix(16)  OutScaling=2^0
  Sine Wave1 : Sin  Frequency=F*2*pi  Phase=PH*pi/180  SampleTime=0
  Sum1 : Sum  Inputs=-+  OutDataType=sfix(16)  OutScaling=2^0
  TonDelay : Subsystem  mask(TonDelay){DT=TD}
      mask prompts: DT "Dead Time"
      mask help: Turn on dead time to protect against short circuit of the converter leg
  XOR : Logic  Operator=XOR
  Out1 : Outport
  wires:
  Fcn/1 -> Sum1/1
  Sine Wave1/1 -> Fcn/1
  XOR/1 -> DT/1
  Relay/1 -> TonDelay/1(s1), DT2/1
  TonDelay/1(s1d) -> DT1/1
  Sum1/1 -> Relay/1
  In1/1 -> Sum1/2
  DT/1 -> Out1/1
  DT1/1 -> XOR/1
  DT2/1 -> XOR/2

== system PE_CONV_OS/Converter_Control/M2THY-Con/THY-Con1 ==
  In1 : Inport  OutDataType=sfix(16)  OutScaling=2^0
  DT : DataTypeConversion
  DT1 : DataTypeConversion
  DT2 : DataTypeConversion
  Fcn : Fcn  Expr="(u  > 0.9999)*2 + (u<=0.9999)*u"
  Relay : Relay  OutDataType=sfix(16)  OutScaling=2^0
  Sine Wave1 : Sin  Frequency=F*2*pi  Phase=PH*pi/180  SampleTime=0
  Sum1 : Sum  Inputs=-+  OutDataType=sfix(16)  OutScaling=2^0
  TonDelay : Subsystem  mask(TonDelay){DT=TD}
      mask prompts: DT "Dead Time"
      mask help: Turn on dead time to protect against short circuit of the converter leg
  XOR : Logic  Operator=XOR
  Out1 : Outport
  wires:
  In1/1 -> Sum1/2
  Sum1/1 -> Relay/1
  TonDelay/1(s1d) -> DT1/1
  Relay/1 -> TonDelay/1(s1), DT2/1
  XOR/1 -> DT/1
  Sine Wave1/1 -> Fcn/1
  Fcn/1 -> Sum1/1
  DT/1 -> Out1/1
  DT1/1 -> XOR/1
  DT2/1 -> XOR/2

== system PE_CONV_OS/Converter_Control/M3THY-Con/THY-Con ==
  In1 : Inport  OutDataType=sfix(16)  OutScaling=2^0
  DT : DataTypeConversion
  DT1 : DataTypeConversion
  DT2 : DataTypeConversion
  Fcn : Fcn  Expr="(u  > 0.9999)*2 + (u<=0.9999)*u"
  Relay : Relay  OutDataType=sfix(16)  OutScaling=2^0
  Sine Wave1 : Sin  Frequency=F*2*pi  Phase=PH*pi/180  SampleTime=0
  Sum1 : Sum  Inputs=-+  OutDataType=sfix(16)  OutScaling=2^0
  TonDelay : Subsystem  mask(TonDelay){DT=TD}
      mask prompts: DT "Dead Time"
      mask help: Turn on dead time to protect against short circuit of the converter leg
  XOR : Logic  Operator=XOR
  Out1 : Outport
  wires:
  In1/1 -> Sum1/2
  Sum1/1 -> Relay/1
  TonDelay/1(s1d) -> DT1/1
  Relay/1 -> TonDelay/1(s1), DT2/1
  XOR/1 -> DT/1
  Sine Wave1/1 -> Fcn/1
  Fcn/1 -> Sum1/1
  DT/1 -> Out1/1
  DT1/1 -> XOR/1
  DT2/1 -> XOR/2

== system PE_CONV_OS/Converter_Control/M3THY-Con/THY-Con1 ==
  In1 : Inport  OutDataType=sfix(16)  OutScaling=2^0
  DT : DataTypeConversion
  DT1 : DataTypeConversion
  DT2 : DataTypeConversion
  Fcn : Fcn  Expr="(u  > 0.9999)*2 + (u<=0.9999)*u"
  Relay : Relay  OutDataType=sfix(16)  OutScaling=2^0
  Sine Wave1 : Sin  Frequency=F*2*pi  Phase=PH*pi/180  SampleTime=0
  Sum1 : Sum  Inputs=-+  OutDataType=sfix(16)  OutScaling=2^0
  TonDelay : Subsystem  mask(TonDelay){DT=TD}
      mask prompts: DT "Dead Time"
      mask help: Turn on dead time to protect against short circuit of the converter leg
  XOR : Logic  Operator=XOR
  Out1 : Outport
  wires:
  Fcn/1 -> Sum1/1
  Sine Wave1/1 -> Fcn/1
  XOR/1 -> DT/1
  Relay/1 -> TonDelay/1(s1), DT2/1
  TonDelay/1(s1d) -> DT1/1
  Sum1/1 -> Relay/1
  In1/1 -> Sum1/2
  DT/1 -> Out1/1
  DT1/1 -> XOR/1
  DT2/1 -> XOR/2

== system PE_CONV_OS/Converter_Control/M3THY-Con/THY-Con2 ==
  In1 : Inport  OutDataType=sfix(16)  OutScaling=2^0
  DT : DataTypeConversion
  DT1 : DataTypeConversion
  DT2 : DataTypeConversion
  Fcn : Fcn  Expr="(u  > 0.9999)*2 + (u<=0.9999)*u"
  Relay : Relay  OutDataType=sfix(16)  OutScaling=2^0
  Sine Wave1 : Sin  Frequency=F*2*pi  Phase=PH*pi/180  SampleTime=0
  Sum1 : Sum  Inputs=-+  OutDataType=sfix(16)  OutScaling=2^0
  TonDelay : Subsystem  mask(TonDelay){DT=TD}
      mask prompts: DT "Dead Time"
      mask help: Turn on dead time to protect against short circuit of the converter leg
  XOR : Logic  Operator=XOR
  Out1 : Outport
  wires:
  In1/1 -> Sum1/2
  Sum1/1 -> Relay/1
  TonDelay/1(s1d) -> DT1/1
  Relay/1 -> TonDelay/1(s1), DT2/1
  XOR/1 -> DT/1
  Sine Wave1/1 -> Fcn/1
  Fcn/1 -> Sum1/1
  DT/1 -> Out1/1
  DT1/1 -> XOR/1
  DT2/1 -> XOR/2

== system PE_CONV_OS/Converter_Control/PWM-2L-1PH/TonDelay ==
  s1 : Inport  Orientation=down  OutDataType=sfix(16)  OutScaling=2^0
  Int : Integrator  ExternalReset=falling
  Rel1 : Relay  OnSwitchValue=DT  OutDataType=sfix(16)  OutScaling=2^0
  s1d : Outport  InitialOutput=0
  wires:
  Rel1/1 -> s1d/1
  s1/1 -> Int/1, Int/2
  Int/1 -> Rel1/1

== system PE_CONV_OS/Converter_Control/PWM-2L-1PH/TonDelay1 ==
  s1 : Inport  Orientation=down  OutDataType=sfix(16)  OutScaling=2^0
  Int : Integrator  ExternalReset=falling
  Rel1 : Relay  OnSwitchValue=DT  OutDataType=sfix(16)  OutScaling=2^0
  s1d : Outport  InitialOutput=0
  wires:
  Rel1/1 -> s1d/1
  s1/1 -> Int/1, Int/2
  Int/1 -> Rel1/1

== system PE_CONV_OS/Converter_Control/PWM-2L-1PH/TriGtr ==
  Clock : Clock
  S2 : Subsystem
  Sum : Sum  OutDataType=sfix(16)  OutScaling=2^0
  T : Constant  Value=T  OutDataType=sfix(16)  OutScaling=2^0
  Td : Constant  Value=Td  OutDataType=sfix(16)  OutScaling=2^0
  mod : Math  Operator=mod
  O : Outport  InitialOutput=0
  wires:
  Td/1 -> Sum/2
  Sum/1 -> mod/1
  T/1 -> mod/2
  Clock/1 -> Sum/1
  S2/1(O1) -> O/1
  mod/1 -> S2/1(I1)

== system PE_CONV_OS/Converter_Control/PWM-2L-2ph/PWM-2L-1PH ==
  In1 : Inport  OutDataType=sfix(16)  OutScaling=2^0
  DT : DataTypeConversion
  DT1 : DataTypeConversion
  Mux : Mux  Inputs=2
  Relay : Relay  OutDataType=sfix(16)  OutScaling=2^0
  Sum : Sum  Inputs=+-  OutDataType=sfix(16)  OutScaling=2^0
  TonDelay : Subsystem  mask(TonDelay){DT=DT}
      mask prompts: DT "Dead Time"
      mask help: Turn on dead time to protect against short circuit of the converter leg
  TonDelay1 : Subsystem  mask(TonDelay){DT=DT}
      mask prompts: DT "Dead Time"
      mask help: Turn on dead time to protect against short circuit of the converter leg
  TriGtr : Subsystem  mask(TriGtr){T=1/FT, Td=PHT/FT/360}
      mask prompts: T "Period Time"; Td "Time Delay"
      mask help: Triangular Wave Generator with variable time delay
  not : Logic  Operator=NOT  Inputs=1
  Out1 : Outport  InitialOutput=0
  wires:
  Mux/1 -> Out1/1
  TonDelay/1(s1d) -> Mux/1
  Relay/1 -> TonDelay/1(s1), DT1/1
  TonDelay1/1(s1d) -> Mux/2
  not/1 -> DT/1
  Sum/1 -> Relay/1
  TriGtr/1(O) -> Sum/2
  In1/1 -> Sum/1
  DT/1 -> TonDelay1/1(s1)
  DT1/1 -> not/1

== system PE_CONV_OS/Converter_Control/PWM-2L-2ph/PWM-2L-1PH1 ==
  In1 : Inport  OutDataType=sfix(16)  OutScaling=2^0
  DT : DataTypeConversion
  DT1 : DataTypeConversion
  Mux : Mux  Inputs=2
  Relay : Relay  OutDataType=sfix(16)  OutScaling=2^0
  Sum : Sum  Inputs=+-  OutDataType=sfix(16)  OutScaling=2^0
  TonDelay : Subsystem  mask(TonDelay){DT=DT}
      mask prompts: DT "Dead Time"
      mask help: Turn on dead time to protect against short circuit of the converter leg
  TonDelay1 : Subsystem  mask(TonDelay){DT=DT}
      mask prompts: DT "Dead Time"
      mask help: Turn on dead time to protect against short circuit of the converter leg
  TriGtr : Subsystem  mask(TriGtr){T=1/FT, Td=PHT/FT/360}
      mask prompts: T "Period Time"; Td "Time Delay"
      mask help: Triangular Wave Generator with variable time delay
  not : Logic  Operator=NOT  Inputs=1
  Out1 : Outport  InitialOutput=0
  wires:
  DT1/1 -> not/1
  DT/1 -> TonDelay1/1(s1)
  In1/1 -> Sum/1
  TriGtr/1(O) -> Sum/2
  Sum/1 -> Relay/1
  not/1 -> DT/1
  TonDelay1/1(s1d) -> Mux/2
  Relay/1 -> DT1/1, TonDelay/1(s1)
  TonDelay/1(s1d) -> Mux/1
  Mux/1 -> Out1/1

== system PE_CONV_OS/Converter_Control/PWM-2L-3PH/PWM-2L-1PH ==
  In1 : Inport  OutDataType=sfix(16)  OutScaling=2^0
  DT : DataTypeConversion
  DT1 : DataTypeConversion
  Mux : Mux  Inputs=2
  Relay : Relay  OutDataType=sfix(16)  OutScaling=2^0
  Sum : Sum  Inputs=+-  OutDataType=sfix(16)  OutScaling=2^0
  TonDelay : Subsystem  mask(TonDelay){DT=DT}
      mask prompts: DT "Dead Time"
      mask help: Turn on dead time to protect against short circuit of the converter leg
  TonDelay1 : Subsystem  mask(TonDelay){DT=DT}
      mask prompts: DT "Dead Time"
      mask help: Turn on dead time to protect against short circuit of the converter leg
  TriGtr : Subsystem  mask(TriGtr){T=1/FT, Td=PHT/FT/360}
      mask prompts: T "Period Time"; Td "Time Delay"
      mask help: Triangular Wave Generator with variable time delay
  not : Logic  Operator=NOT  Inputs=1
  Out1 : Outport  InitialOutput=0
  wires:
  DT1/1 -> not/1
  DT/1 -> TonDelay1/1(s1)
  In1/1 -> Sum/1
  TriGtr/1(O) -> Sum/2
  Sum/1 -> Relay/1
  not/1 -> DT/1
  TonDelay1/1(s1d) -> Mux/2
  Relay/1 -> DT1/1, TonDelay/1(s1)
  TonDelay/1(s1d) -> Mux/1
  Mux/1 -> Out1/1

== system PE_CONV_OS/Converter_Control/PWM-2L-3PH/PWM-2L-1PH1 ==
  In1 : Inport  OutDataType=sfix(16)  OutScaling=2^0
  DT : DataTypeConversion
  DT1 : DataTypeConversion
  Mux : Mux  Inputs=2
  Relay : Relay  OutDataType=sfix(16)  OutScaling=2^0
  Sum : Sum  Inputs=+-  OutDataType=sfix(16)  OutScaling=2^0
  TonDelay : Subsystem  mask(TonDelay){DT=DT}
      mask prompts: DT "Dead Time"
      mask help: Turn on dead time to protect against short circuit of the converter leg
  TonDelay1 : Subsystem  mask(TonDelay){DT=DT}
      mask prompts: DT "Dead Time"
      mask help: Turn on dead time to protect against short circuit of the converter leg
  TriGtr : Subsystem  mask(TriGtr){T=1/FT, Td=PHT/FT/360}
      mask prompts: T "Period Time"; Td "Time Delay"
      mask help: Triangular Wave Generator with variable time delay
  not : Logic  Operator=NOT  Inputs=1
  Out1 : Outport  InitialOutput=0
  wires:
  Mux/1 -> Out1/1
  TonDelay/1(s1d) -> Mux/1
  Relay/1 -> TonDelay/1(s1), DT1/1
  TonDelay1/1(s1d) -> Mux/2
  not/1 -> DT/1
  Sum/1 -> Relay/1
  TriGtr/1(O) -> Sum/2
  In1/1 -> Sum/1
  DT/1 -> TonDelay1/1(s1)
  DT1/1 -> not/1

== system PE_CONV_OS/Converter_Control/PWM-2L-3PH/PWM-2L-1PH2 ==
  In1 : Inport  OutDataType=sfix(16)  OutScaling=2^0
  DT : DataTypeConversion
  DT1 : DataTypeConversion
  Mux : Mux  Inputs=2
  Relay : Relay  OutDataType=sfix(16)  OutScaling=2^0
  Sum : Sum  Inputs=+-  OutDataType=sfix(16)  OutScaling=2^0
  TonDelay : Subsystem  mask(TonDelay){DT=DT}
      mask prompts: DT "Dead Time"
      mask help: Turn on dead time to protect against short circuit of the converter leg
  TonDelay1 : Subsystem  mask(TonDelay){DT=DT}
      mask prompts: DT "Dead Time"
      mask help: Turn on dead time to protect against short circuit of the converter leg
  TriGtr : Subsystem  mask(TriGtr){T=1/FT, Td=PHT/FT/360}
      mask prompts: T "Period Time"; Td "Time Delay"
      mask help: Triangular Wave Generator with variable time delay
  not : Logic  Operator=NOT  Inputs=1
  Out1 : Outport  InitialOutput=0
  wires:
  DT1/1 -> not/1
  DT/1 -> TonDelay1/1(s1)
  In1/1 -> Sum/1
  TriGtr/1(O) -> Sum/2
  Sum/1 -> Relay/1
  not/1 -> DT/1
  TonDelay1/1(s1d) -> Mux/2
  Relay/1 -> DT1/1, TonDelay/1(s1)
  TonDelay/1(s1d) -> Mux/1
  Mux/1 -> Out1/1

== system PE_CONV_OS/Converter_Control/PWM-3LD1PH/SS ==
  I1 : Inport  OutDataType=sfix(16)  OutScaling=2^0
  DT : DataTypeConversion
  DT1 : DataTypeConversion
  Relay : Relay  OutDataType=sfix(16)  OutScaling=2^0
  Sum : Sum  Inputs=+-  OutDataType=sfix(16)  OutScaling=2^0
  TonDelay : Subsystem  mask(TonDelay){DT=DT}
      mask prompts: DT "Dead Time"
      mask help: Turn on dead time to protect against short circuit of the converter leg
  TonDelay1 : Subsystem  mask(TonDelay){DT=DT}
      mask prompts: DT "Dead Time"
      mask help: Turn on dead time to protect against short circuit of the converter leg
  TriGtr-AO : Subsystem  mask(TriGtr-AO){A=A, O=O1, T=1/FT, Td=PHT/FT/180}
      mask prompts: A "Amplitude"; O "Offset"; T "Period Time"; Td "Time Delay"
      mask help: Triangular Wave Generator with variable time delay, variable amplitude and offset
  not : Logic  Operator=NOT  Inputs=1
  O1 : Outport  InitialOutput=0
  O2 : Outport  Port=2  InitialOutput=0
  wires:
  TonDelay/1(s1d) -> O1/1
  Relay/1 -> TonDelay/1(s1), DT1/1
  TonDelay1/1(s1d) -> O2/1
  not/1 -> DT/1
  Sum/1 -> Relay/1
  TriGtr-AO/1(Out1) -> Sum/2
  I1/1 -> Sum/1
  DT/1 -> TonDelay1/1(s1)
  DT1/1 -> not/1

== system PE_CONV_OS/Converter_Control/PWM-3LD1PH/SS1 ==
  I1 : Inport  OutDataType=sfix(16)  OutScaling=2^0
  DT : DataTypeConversion
  DT1 : DataTypeConversion
  Relay : Relay  OutDataType=sfix(16)  OutScaling=2^0
  Sum : Sum  Inputs=+-  OutDataType=sfix(16)  OutScaling=2^0
  TonDelay : Subsystem  mask(TonDelay){DT=DT}
      mask prompts: DT "Dead Time"
      mask help: Turn on dead time to protect against short circuit of the converter leg
  TonDelay1 : Subsystem  mask(TonDelay){DT=DT}
      mask prompts: DT "Dead Time"
      mask help: Turn on dead time to protect against short circuit of the converter leg
  TriGtr-AO : Subsystem  mask(TriGtr-AO){A=A, O=O2, T=1/FT, Td=PHT/FT/180}
      mask prompts: A "Amplitude"; O "Offset"; T "Period Time"; Td "Time Delay"
      mask help: Triangular Wave Generator with variable time delay, variable amplitude and offset
  not : Logic  Operator=NOT  Inputs=1
  O1 : Outport  InitialOutput=0
  O2 : Outport  Port=2  InitialOutput=0
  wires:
  TonDelay/1(s1d) -> O1/1
  Relay/1 -> TonDelay/1(s1), DT1/1
  TonDelay1/1(s1d) -> O2/1
  not/1 -> DT/1
  Sum/1 -> Relay/1
  TriGtr-AO/1(Out1) -> Sum/2
  I1/1 -> Sum/1
  DT/1 -> TonDelay1/1(s1)
  DT1/1 -> not/1

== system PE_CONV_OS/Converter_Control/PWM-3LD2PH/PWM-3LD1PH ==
  In1 : Inport  OutDataType=sfix(16)  OutScaling=2^0
  Mux : Mux
  SS : Subsystem
  SS1 : Subsystem
  Out1 : Outport
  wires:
  SS1/2(O2) -> Mux/4
  SS/1(O1) -> Mux/1
  Mux/1 -> Out1/1
  SS/2(O2) -> Mux/3
  SS1/1(O1) -> Mux/2
  In1/1 -> SS/1(I1), SS1/1(I1)

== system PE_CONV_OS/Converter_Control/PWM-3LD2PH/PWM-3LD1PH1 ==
  In1 : Inport  OutDataType=sfix(16)  OutScaling=2^0
  Mux : Mux
  SS : Subsystem
  SS1 : Subsystem
  Out1 : Outport
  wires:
  In1/1 -> SS1/1(I1), SS/1(I1)
  SS1/1(O1) -> Mux/2
  SS/2(O2) -> Mux/3
  Mux/1 -> Out1/1
  SS/1(O1) -> Mux/1
  SS1/2(O2) -> Mux/4

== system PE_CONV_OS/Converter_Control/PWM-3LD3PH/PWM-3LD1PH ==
  In1 : Inport  OutDataType=sfix(16)  OutScaling=2^0
  Mux : Mux
  SS : Subsystem
  SS1 : Subsystem
  Out1 : Outport
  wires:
  SS1/2(O2) -> Mux/4
  SS/1(O1) -> Mux/1
  Mux/1 -> Out1/1
  SS/2(O2) -> Mux/3
  SS1/1(O1) -> Mux/2
  In1/1 -> SS/1(I1), SS1/1(I1)

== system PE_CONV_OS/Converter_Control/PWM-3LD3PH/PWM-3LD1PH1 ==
  In1 : Inport  OutDataType=sfix(16)  OutScaling=2^0
  Mux : Mux
  SS : Subsystem
  SS1 : Subsystem
  Out1 : Outport
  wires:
  In1/1 -> SS1/1(I1), SS/1(I1)
  SS1/1(O1) -> Mux/2
  SS/2(O2) -> Mux/3
  Mux/1 -> Out1/1
  SS/1(O1) -> Mux/1
  SS1/2(O2) -> Mux/4

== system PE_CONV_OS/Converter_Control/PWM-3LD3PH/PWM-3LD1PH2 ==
  In1 : Inport  OutDataType=sfix(16)  OutScaling=2^0
  Mux : Mux
  SS : Subsystem
  SS1 : Subsystem
  Out1 : Outport
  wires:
  SS1/2(O2) -> Mux/4
  SS/1(O1) -> Mux/1
  Mux/1 -> Out1/1
  SS/2(O2) -> Mux/3
  SS1/1(O1) -> Mux/2
  In1/1 -> SS/1(I1), SS1/1(I1)

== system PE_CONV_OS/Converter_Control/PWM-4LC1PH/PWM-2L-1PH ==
  In1 : Inport  OutDataType=sfix(16)  OutScaling=2^0
  DT : DataTypeConversion
  DT1 : DataTypeConversion
  Relay : Relay  OutDataType=sfix(16)  OutScaling=2^0
  Sum : Sum  Inputs=+-  OutDataType=sfix(16)  OutScaling=2^0
  TonDelay : Subsystem  mask(TonDelay){DT=DT}
      mask prompts: DT "Dead Time"
      mask help: Turn on dead time to protect against short circuit of the converter leg
  TonDelay1 : Subsystem  mask(TonDelay){DT=DT}
      mask prompts: DT "Dead Time"
      mask help: Turn on dead time to protect against short circuit of the converter leg
  TriGtr : Subsystem  mask(TriGtr){T=1/FT, Td=PHT/FT/360}
      mask prompts: T "Period Time"; Td "Time Delay"
      mask help: Triangular Wave Generator with variable time delay
  not : Logic  Operator=NOT  Inputs=1
  Out1 : Outport  InitialOutput=0
  Out2 : Outport  Port=2  InitialOutput=0
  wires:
  TonDelay/1(s1d) -> Out1/1
  Relay/1 -> TonDelay/1(s1), DT1/1
  TonDelay1/1(s1d) -> Out2/1
  not/1 -> DT/1
  Sum/1 -> Relay/1
  TriGtr/1(O) -> Sum/2
  In1/1 -> Sum/1
  DT/1 -> TonDelay1/1(s1)
  DT1/1 -> not/1

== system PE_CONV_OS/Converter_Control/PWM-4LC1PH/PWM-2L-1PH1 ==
  In1 : Inport  OutDataType=sfix(16)  OutScaling=2^0
  DT : DataTypeConversion
  DT1 : DataTypeConversion
  Relay : Relay  OutDataType=sfix(16)  OutScaling=2^0
  Sum : Sum  Inputs=+-  OutDataType=sfix(16)  OutScaling=2^0
  TonDelay : Subsystem  mask(TonDelay){DT=DT}
      mask prompts: DT "Dead Time"
      mask help: Turn on dead time to protect against short circuit of the converter leg
  TonDelay1 : Subsystem  mask(TonDelay){DT=DT}
      mask prompts: DT "Dead Time"
      mask help: Turn on dead time to protect against short circuit of the converter leg
  TriGtr : Subsystem  mask(TriGtr){T=1/FT, Td=PHT/FT/360}
      mask prompts: T "Period Time"; Td "Time Delay"
      mask help: Triangular Wave Generator with variable time delay
  not : Logic  Operator=NOT  Inputs=1
  Out1 : Outport  InitialOutput=0
  Out2 : Outport  Port=2  InitialOutput=0
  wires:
  DT1/1 -> not/1
  DT/1 -> TonDelay1/1(s1)
  In1/1 -> Sum/1
  TriGtr/1(O) -> Sum/2
  Sum/1 -> Relay/1
  not/1 -> DT/1
  TonDelay1/1(s1d) -> Out2/1
  Relay/1 -> DT1/1, TonDelay/1(s1)
  TonDelay/1(s1d) -> Out1/1

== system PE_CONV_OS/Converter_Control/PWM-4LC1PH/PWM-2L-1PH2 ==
  In1 : Inport  OutDataType=sfix(16)  OutScaling=2^0
  DT : DataTypeConversion
  DT1 : DataTypeConversion
  Relay : Relay  OutDataType=sfix(16)  OutScaling=2^0
  Sum : Sum  Inputs=+-  OutDataType=sfix(16)  OutScaling=2^0
  TonDelay : Subsystem  mask(TonDelay){DT=DT}
      mask prompts: DT "Dead Time"
      mask help: Turn on dead time to protect against short circuit of the converter leg
  TonDelay1 : Subsystem  mask(TonDelay){DT=DT}
      mask prompts: DT "Dead Time"
      mask help: Turn on dead time to protect against short circuit of the converter leg
  TriGtr : Subsystem  mask(TriGtr){T=1/FT, Td=PHT/FT/360}
      mask prompts: T "Period Time"; Td "Time Delay"
      mask help: Triangular Wave Generator with variable time delay
  not : Logic  Operator=NOT  Inputs=1
  Out1 : Outport  InitialOutput=0
  Out2 : Outport  Port=2  InitialOutput=0
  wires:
  TonDelay/1(s1d) -> Out1/1
  Relay/1 -> TonDelay/1(s1), DT1/1
  TonDelay1/1(s1d) -> Out2/1
  not/1 -> DT/1
  Sum/1 -> Relay/1
  TriGtr/1(O) -> Sum/2
  In1/1 -> Sum/1
  DT/1 -> TonDelay1/1(s1)
  DT1/1 -> not/1

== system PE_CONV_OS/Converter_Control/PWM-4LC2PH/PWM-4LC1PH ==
  In1 : Inport  OutDataType=sfix(16)  OutScaling=2^0
  Mux : Mux  Inputs=6
  PWM-2L-1PH : Subsystem  mask(PWM-2L-1PH){FT=FT, PHT=PHT1, DT=DT}
      mask prompts: FT "Triangular Frequency"; PHT "Trian. Phase Angle (Degree)"; DT "Dead Time"
      mask help: Pulse Width Modulation for 1 Phase Converter
  PWM-2L-1PH1 : Subsystem  mask(PWM-2L-1PH){FT=FT, PHT=PHT2, DT=DT}
      mask prompts: FT "Triangular Frequency"; PHT "Trian. Phase Angle (Degree)"; DT "Dead Time"
      mask help: Pulse Width Modulation for 1 Phase Converter
  PWM-2L-1PH2 : Subsystem  mask(PWM-2L-1PH){FT=FT, PHT=PHT3, DT=DT}
      mask prompts: FT "Triangular Frequency"; PHT "Trian. Phase Angle (Degree)"; DT "Dead Time"
      mask help: Pulse Width Modulation for 1 Phase Converter
  Out1 : Outport
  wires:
  PWM-2L-1PH/2(Out2) -> Mux/6
  In1/1 -> PWM-2L-1PH2/1(In1), PWM-2L-1PH1/1(In1), PWM-2L-1PH/1(In1)
  Mux/1 -> Out1/1
  PWM-2L-1PH2/2(Out2) -> Mux/4
  PWM-2L-1PH2/1(Out1) -> Mux/3
  PWM-2L-1PH1/2(Out2) -> Mux/5
  PWM-2L-1PH1/1(Out1) -> Mux/2
  PWM-2L-1PH/1(Out1) -> Mux/1

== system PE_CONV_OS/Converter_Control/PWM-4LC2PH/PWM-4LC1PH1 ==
  In1 : Inport  OutDataType=sfix(16)  OutScaling=2^0
  Mux : Mux  Inputs=6
  PWM-2L-1PH : Subsystem  mask(PWM-2L-1PH){FT=FT, PHT=PHT1, DT=DT}
      mask prompts: FT "Triangular Frequency"; PHT "Trian. Phase Angle (Degree)"; DT "Dead Time"
      mask help: Pulse Width Modulation for 1 Phase Converter
  PWM-2L-1PH1 : Subsystem  mask(PWM-2L-1PH){FT=FT, PHT=PHT2, DT=DT}
      mask prompts: FT "Triangular Frequency"; PHT "Trian. Phase Angle (Degree)"; DT "Dead Time"
      mask help: Pulse Width Modulation for 1 Phase Converter
  PWM-2L-1PH2 : Subsystem  mask(PWM-2L-1PH){FT=FT, PHT=PHT3, DT=DT}
      mask prompts: FT "Triangular Frequency"; PHT "Trian. Phase Angle (Degree)"; DT "Dead Time"
      mask help: Pulse Width Modulation for 1 Phase Converter
  Out1 : Outport
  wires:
  PWM-2L-1PH/1(Out1) -> Mux/1
  PWM-2L-1PH1/1(Out1) -> Mux/2
  PWM-2L-1PH1/2(Out2) -> Mux/5
  PWM-2L-1PH2/1(Out1) -> Mux/3
  PWM-2L-1PH2/2(Out2) -> Mux/4
  Mux/1 -> Out1/1
  In1/1 -> PWM-2L-1PH/1(In1), PWM-2L-1PH1/1(In1), PWM-2L-1PH2/1(In1)
  PWM-2L-1PH/2(Out2) -> Mux/6

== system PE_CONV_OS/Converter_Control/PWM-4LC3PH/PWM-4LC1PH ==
  In1 : Inport  OutDataType=sfix(16)  OutScaling=2^0
  Mux : Mux  Inputs=6
  PWM-2L-1PH : Subsystem  mask(PWM-2L-1PH){FT=FT, PHT=PHT1, DT=DT}
      mask prompts: FT "Triangular Frequency"; PHT "Trian. Phase Angle (Degree)"; DT "Dead Time"
      mask help: Pulse Width Modulation for 1 Phase Converter
  PWM-2L-1PH1 : Subsystem  mask(PWM-2L-1PH){FT=FT, PHT=PHT2, DT=DT}
      mask prompts: FT "Triangular Frequency"; PHT "Trian. Phase Angle (Degree)"; DT "Dead Time"
      mask help: Pulse Width Modulation for 1 Phase Converter
  PWM-2L-1PH2 : Subsystem  mask(PWM-2L-1PH){FT=FT, PHT=PHT3, DT=DT}
      mask prompts: FT "Triangular Frequency"; PHT "Trian. Phase Angle (Degree)"; DT "Dead Time"
      mask help: Pulse Width Modulation for 1 Phase Converter
  Out1 : Outport
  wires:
  PWM-2L-1PH/2(Out2) -> Mux/6
  In1/1 -> PWM-2L-1PH/1(In1), PWM-2L-1PH1/1(In1), PWM-2L-1PH2/1(In1)
  Mux/1 -> Out1/1
  PWM-2L-1PH2/2(Out2) -> Mux/4
  PWM-2L-1PH2/1(Out1) -> Mux/3
  PWM-2L-1PH1/2(Out2) -> Mux/5
  PWM-2L-1PH1/1(Out1) -> Mux/2
  PWM-2L-1PH/1(Out1) -> Mux/1

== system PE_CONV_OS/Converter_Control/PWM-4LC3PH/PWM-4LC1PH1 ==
  In1 : Inport  OutDataType=sfix(16)  OutScaling=2^0
  Mux : Mux  Inputs=6
  PWM-2L-1PH : Subsystem  mask(PWM-2L-1PH){FT=FT, PHT=PHT1, DT=DT}
      mask prompts: FT "Triangular Frequency"; PHT "Trian. Phase Angle (Degree)"; DT "Dead Time"
      mask help: Pulse Width Modulation for 1 Phase Converter
  PWM-2L-1PH1 : Subsystem  mask(PWM-2L-1PH){FT=FT, PHT=PHT2, DT=DT}
      mask prompts: FT "Triangular Frequency"; PHT "Trian. Phase Angle (Degree)"; DT "Dead Time"
      mask help: Pulse Width Modulation for 1 Phase Converter
  PWM-2L-1PH2 : Subsystem  mask(PWM-2L-1PH){FT=FT, PHT=PHT3, DT=DT}
      mask prompts: FT "Triangular Frequency"; PHT "Trian. Phase Angle (Degree)"; DT "Dead Time"
      mask help: Pulse Width Modulation for 1 Phase Converter
  Out1 : Outport
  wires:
  PWM-2L-1PH/1(Out1) -> Mux/1
  PWM-2L-1PH1/1(Out1) -> Mux/2
  PWM-2L-1PH1/2(Out2) -> Mux/5
  PWM-2L-1PH2/1(Out1) -> Mux/3
  PWM-2L-1PH2/2(Out2) -> Mux/4
  Mux/1 -> Out1/1
  In1/1 -> PWM-2L-1PH2/1(In1), PWM-2L-1PH1/1(In1), PWM-2L-1PH/1(In1)
  PWM-2L-1PH/2(Out2) -> Mux/6
